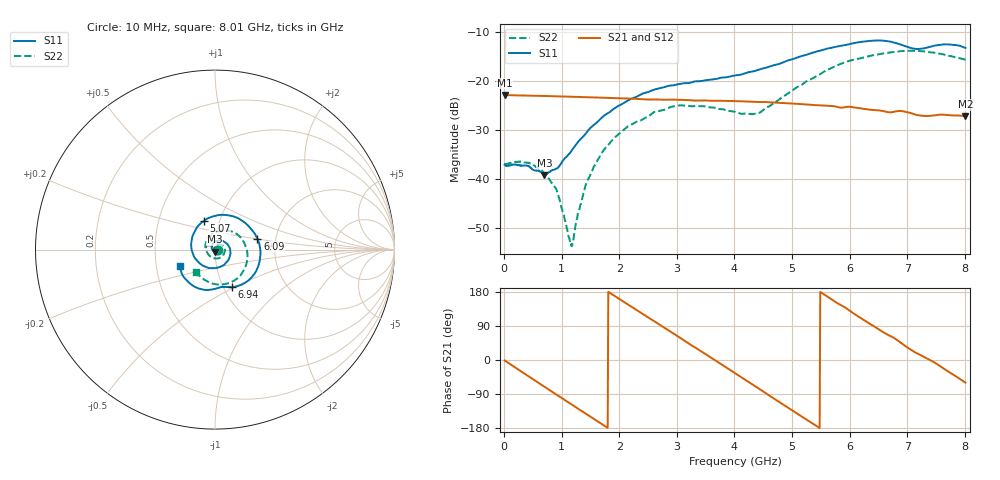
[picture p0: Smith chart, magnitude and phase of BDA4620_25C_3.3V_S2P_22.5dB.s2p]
!Agilent Technologies,E5071B,MY42404982,A.09.10
!Date: Wed May 06 08:53:40 2026
!Data & Calibration Information:
!Freq	S11:SOLT2(ON)	S21:SOLT2(ON)	S12:SOLT2(ON)	S22:SOLT2(ON)
# Hz S RI R 50
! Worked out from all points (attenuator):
!   801 points, 10 MHz to 8.01 GHz, reference 50 ohm
!   highest |S21| = -22.89 dB at 10 MHz (marker M1); lowest = -27.3 dB at 8.01 GHz (marker M2)
!   lowest |S11| = -39.2 dB at 700 MHz (marker M3), VSWR 1.02, Z = 49.8 - j1.08 ohm
!   |S11| at or under -10 dB: start of sweep to end of sweep
!   |S22| runs from -53.8 to -13.8 dB; largest |S21 - S12| = 0.00028
!   S11 on the Smith chart (normalised r, x): 10 MHz: 1.03, -0.00; 5.07 GHz: 0.84, +0.28; 6.09 GHz: 1.60, +0.21; 6.94 GHz: 1.10, -0.48; 8.01 GHz: 0.66, -0.13
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1e7  0.0139 -0.000928  0.0717 -0.0015  0.0718 -0.00151  0.0141 -0.000471
4.2e8  0.00891 -0.0101  0.0521 -0.0476  0.0522 -0.0477  0.0136 -0.00501
7e8  -0.00148 -0.0109  0.0235 -0.0659  0.0235 -0.0661  0.00894 -0.00717
9.2e8  -0.0111 -0.00625  -0.00273 -0.0694  -0.0028 -0.0695  0.00364 -0.00648
1.16e9  -0.0178 0.00612  -0.0302 -0.0618  -0.0304 -0.0618  -0.00171 -0.00118
1.2e9  -0.0184 0.00862  -0.0344 -0.0594  -0.0345 -0.0595  -0.0023 2.35e-05
1.35e9  -0.0183 0.0186  -0.0482 -0.0484  -0.0482 -0.0484  -0.00381 0.00465
1.53e9  -0.0133 0.0316  -0.0601 -0.0312  -0.0602 -0.0312  -0.00368 0.0114
1.77e9  0.00176 0.0453  -0.0669 -0.0045  -0.0671 -0.00443  0.000604 0.0208
2.15e9  0.0393 0.0491  -0.055 0.0365  -0.055 0.0366  0.0172 0.0296
2.68e9  0.0833 0.00465  -0.00585 0.0641  -0.00584 0.0642  0.0448 0.0196
3.08e9  0.0765 -0.0541  0.0355 0.0531  0.0357 0.0531  0.0557 -0.0076
4.01e9  -0.0773 -0.0832  0.0509 -0.0354  0.051 -0.0356  -0.0108 -0.047
4.42e9  -0.13 -0.00139  0.0156 -0.0588  0.0156 -0.0589  -0.0451 -0.0129
5.07e9  -0.0633 0.1592  -0.0443 -0.0379  -0.0444 -0.038  -0.0231 0.0816
5.35e9  0.0206 0.1923  -0.0553 -0.0129  -0.0554 -0.0129  0.023 0.1029
6.09e9  0.2359 0.0614  -0.0271 0.0459  -0.0272 0.046  0.1593 0.0443
6.39e9  0.2493 -0.0629  -0.00176 0.0504  -0.00177 0.0505  0.1805 -0.0213
6.68e9  0.1853 -0.1728  0.02 0.0433  0.0201 0.0434  0.1711 -0.0913
6.94e9  0.0944 -0.2085  0.0375 0.031  0.0376 0.031  0.1374 -0.1486
7.58e9  -0.0796 -0.2199  0.0431 -0.0134  0.0432 -0.0133  -0.0195 -0.1874
8.01e9  -0.1956 -0.094  0.0219 -0.0374  0.0219 -0.0375  -0.1032 -0.1272
